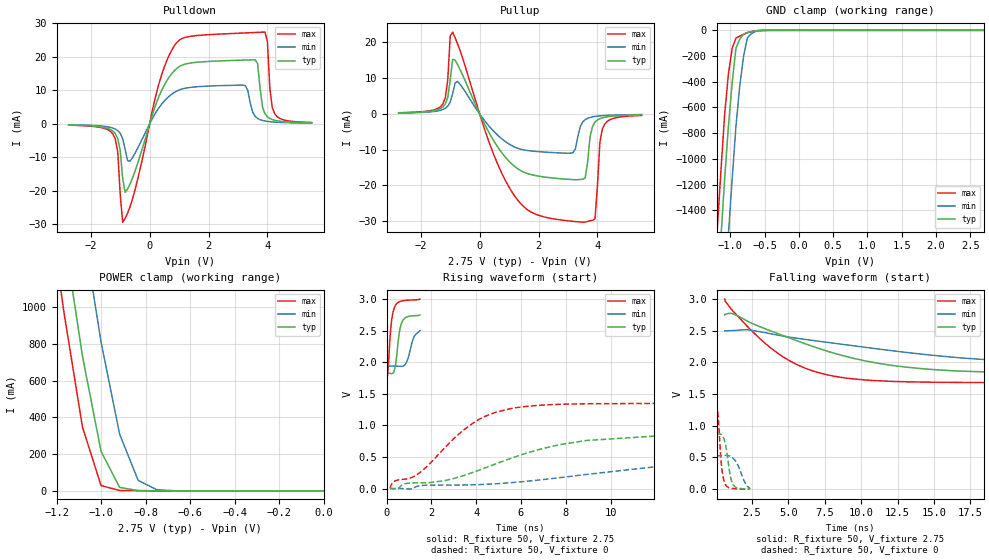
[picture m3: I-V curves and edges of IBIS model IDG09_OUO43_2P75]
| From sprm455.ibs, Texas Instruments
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|   Model Cell IDG09_OUO43_2P75
|IDG09_OUO43_2P75
[Model]   IDG09_OUO43_2P75
Model_type   I/O
Polarity   Non-Inverting
Enable   Active-Low
Vinl =  0.7V
Vinh =  1.7V
Cref =  15pF
Rref =  100.00M
Vref =  0V
Vmeas =  1.375
C_comp   3.134p   3.082p   3.207p
[Model Spec]
Vinl   0.7V   0.7V   0.7V
Vinh   1.7V   1.7V   1.7V
[Temperature Range]   25   125   -40
[Voltage Range]   2.75   2.5   3
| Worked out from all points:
|   slope of the pulldown table from 0 to 0.412 V, typ, clamps not added: 41 ohm
|   slope of the pullup table from 0 to 0.412 V, typ, clamps not added: 62.6 ohm
|   GND clamp passes 1 mA (typ) near -0.54 V on its own axis
|   POWER clamp passes 1 mA (typ) near -0.78 V on its own axis
|   rising waveform, R_fixture 50, V_fixture 2.75: 20-80 % time 203ps typ, 261ps min, 178ps max; typ from 1.82 V to 2.75 V
|   rising waveform, R_fixture 50, V_fixture 0: 20-80 % time 4.55ns typ, 8.74ns min, 2.51ns max; typ from 0 V to 0.861 V
|   falling waveform, R_fixture 50, V_fixture 2.75: 20-80 % time 7.57ns typ, 12.7ns min, 4.29ns max; typ from 2.75 V to 1.82 V
|   falling waveform, R_fixture 50, V_fixture 0: 20-80 % time 352ps typ, 574ps min, 258ps max; typ from 0.861 V to 0 V
[POWER_clamp]
|   voltage   I(typ)   I(min)   I(max)
-2.75V    16.6A      17.26A     16.24A
-1.194V   1.641A     2.388A     1.212A
-1.167V   1.399A     2.143A     971.7mA
-1.139V   1.177A     1.911A     763.3mA
-1.111V   954.7mA    1.678A     555mA
-1.083V   732.5mA    1.445A     346.6mA
-1.056V   560.1mA    1.234A     240.8mA
-1.028V   387.7mA    1.022A     134.9mA
-1V       215.3mA    810.7mA    29.08mA
-916.7mV  19.29mA    309mA      2.477mA
-833.3mV  1.74mA     57.42mA    1.347mA
0V        51.99pA    8.229nA    612.8fA
[Pulldown]
|   voltage   I(typ)   I(min)   I(max)
-2.75V    -360.3uA   -277.2uA   -400.9uA
-1.25V    -2.159mA   -1.266mA   -3.017mA
-1.083V   -4.39mA    -2.026mA   -8.402mA
-916.7mV  -16.29mA   -4.388mA   -29.32mA
-666.7mV  -17.96mA   -11.14mA   -24.73mA
333.3mV   8.511mA    4.998mA    12.5mA
1.083V    17.41mA    10.32mA    25.36mA
3.25V     19.01mA    11.37mA    27.08mA
3.583V    19.04mA    2.232mA    27.22mA
3.917V    2.992mA    841.3uA    27.33mA
4.25V     1.053mA    505.4uA    2.946mA
5.5V      292.8uA    198.8uA    397.1uA
[Pullup]
|   voltage   I(typ)   I(min)   I(max)
-2.75V    285.7uA    234.9uA    326.2uA
-1.25V    1.953mA    1.223mA    2.77mA
-1.083V   4.622mA    2.158mA    9.492mA
-916.7mV  15.25mA    5.649mA    22.87mA
-750mV    13.77mA    9.086mA    19.58mA
1.167V    -14.54mA   -9.171mA   -22.68mA
3.167V    -18.37mA   -10.85mA   -30.03mA
3.5V      -18.26mA   -2.273mA   -30.27mA
3.917V    -2.311mA   -709.8uA   -29.33mA
4.083V    -1.338mA   -549.5uA   -7.934mA
4.25V     -931.1uA   -447.3uA   -2.817mA
5.5V      -276.8uA   -184.6uA   -431.1uA
[GND_clamp]
|   voltage   I(typ)   I(min)   I(max)
-2.75V    -17.13A    -17.98A    -16.66A
-1.194V   -2.125A    -3.035A    -1.593A
-1.139V   -1.641A    -2.542A    -1.12A
-1.083V   -1.169A    -2.057A    -667.5mA
-1.028V   -753mA     -1.596A    -343.2mA
-972.2mV  -409.2mA   -1.159A    -140.9mA
-916.7mV  -137.5mA   -745.4mA   -60.68mA
-861.1mV  -69.45mA   -430.6mA   -44.79mA
-805.6mV  -29.34mA   -201.1mA   -30.93mA
-750mV    -17.2mA    -56.94mA   -19.11mA
-583.3mV  -1.931mA   -3.669mA   -1.173mA
2.694V    50.22pA    162.7nA    435.2fA
[Ramp]
| variable   typ   min   max
dV/dt_f  0.5696523/7.6633119n 0.34558798/12.752003n 0.81181624/4.3298596n
dV/dt_r 0.52264699/4.591718n  0.32063462/8.7223675n 0.81532466/2.5240087n
R_load = 50
[Rising Waveform]
R_fixture = 50
V_fixture = 2.75
V_fixture_min = 2.5
V_fixture_max = 3
|   time   V(typ)   V(min)   V(max)
0s        1.825V     1.939V     1.682V
68.93ps   1.825V     1.939V     1.885V
199.2ps   1.821V     1.94V      2.573V
346.9ps   1.869V     1.939V     2.86V
427.5ps   2.023V     1.938V     2.915V
569.6ps   2.465V     1.936V     2.956V
693.7ps   2.637V     1.935V     2.971V
913.4ps   2.717V     2.017V     2.981V
1.225ns   2.736V     2.398V     2.987V
1.491ns   2.75V      2.5V       3V
[Rising Waveform]
R_fixture = 50
V_fixture = 0
V_fixture_min = 0
V_fixture_max = 0
|   time   V(typ)   V(min)   V(max)
156.2ps   56.03pV    15.9nV     1.153pV
379.3ps   -7.139mV   194.9uV    119.7mV
828.6ps   76.95mV    -2.506mV   149mV
1.483ns   90.84mV    45.05mV    250.4mV
2.582ns   123.8mV    54.74mV    639mV
3.97ns    269.6mV    60.27mV    1.062V
5.634ns   488.9mV    95.39mV    1.272V
8.904ns   759.9mV    222.4mV    1.343V
15.53ns   856.5mV    442.2mV    1.348V
21.47ns   861.2mV    526.4mV    1.348V
[Falling Waveform]
R_fixture = 50
V_fixture = 2.75
V_fixture_min = 2.5
V_fixture_max = 3
|   time   V(typ)   V(min)   V(max)
630.6ps   2.75V      2.5V       3V
1.149ns   2.772V     2.502V     2.824V
2.255ns   2.645V     2.514V     2.553V
4.029ns   2.476V     2.442V     2.186V
5.663ns   2.336V     2.379V     1.958V
7.311ns   2.204V     2.328V     1.824V
10.35ns   2.021V     2.236V     1.722V
14.15ns   1.902V     2.131V     1.69V
19.31ns   1.845V     2.032V     1.683V
25.63ns   1.825V     1.939V     1.682V
[Falling Waveform]
R_fixture = 50
V_fixture = 0
V_fixture_min = 0
V_fixture_max = 0
|   time   V(typ)   V(min)   V(max)
69.92ps   861.2mV    526.4mV    1.348V
189.6ps   868.7mV    526.5mV    1.13V
352.3ps   868.3mV    529.2mV    534.3mV
419ps     858.7mV    530.4mV    353.1mV
634.1ps   754mV      533.7mV    97.81mV
1.011ns   215.5mV    518.8mV    15.85mV
1.181ns   82.69mV    493.8mV    10.04mV
1.521ns   17.8mV     386.7mV    5.535mV
2.04ns    5.175mV    94.32mV    2.637mV
2.373ns   56.03pV    15.9nV     1.153pV
